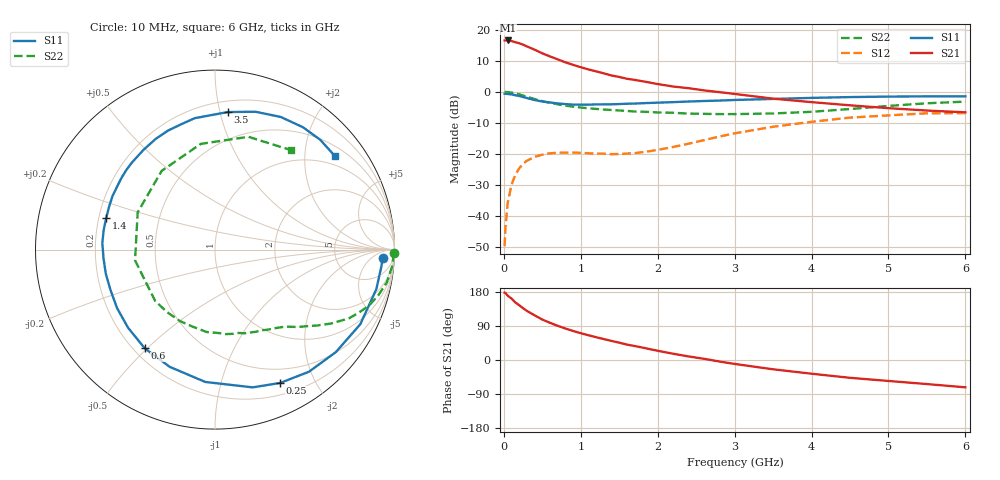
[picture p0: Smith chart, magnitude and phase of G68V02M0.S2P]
! SIEMENS Small Signal Semiconductors
! BFG193
! Si NPN RF Bipolar Junction Transistor in SOT223
! VCE = 8 V  IC = 2 mA
! Common Emitter S-Parameters:  August  1996
# GHz  S  MA  R  50
!  f  S11  S21  S12  S22
! GHz  MAG  ANG  MAG  ANG  MAG  ANG  MAG  ANG
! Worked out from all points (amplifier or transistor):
!   36 points, 10 MHz to 6 GHz, reference 50 ohm
!   highest |S21| = 16.5 dB at 50 MHz (marker M1)
!   |S21| within 3 dB of that: start of sweep to 402.1 MHz
!   unconditionally stable (mu >= 1): 1.376 GHz to 2.522 GHz
!   at 250 MHz: K = 0.17, MSG = 19.1 dB, |S12| = -23.1 dB
!   at 1.4 GHz: K = 1.02, MAG = 11.7 dB, |S12| = -20.0 dB
!   at 6 GHz: K = 0.94, MSG = 0.1 dB, |S12| = -6.8 dB
!   S11 on the Smith chart (normalised r, x): 10 MHz: 19, -14; 250 MHz: 0.33, -1.55; 600 MHz: 0.24, -0.49; 1.4 GHz: 0.23, +0.14; 3.5 GHz: 0.28, +1.06; 6 GHz: 0.74, +2.72
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0.01  0.9345 -2.8  6.709 177.8  0.0033 92.7  0.9971 -1.1
0.02  0.9321 -5.6  6.712 177.0  0.0064 86.3  0.9951 -2.2
0.05  0.9255 -13.8  6.713 169.8  0.0164 82.5  0.9909 -5.5
0.1  0.9101 -27.2  6.557 162.0  0.0321 75.4  0.9746 -10.8
0.15  0.8829 -40.3  6.29 151.9  0.0469 67.2  0.9446 -15.7
0.25  0.827 -63.9  5.748 136.6  0.07 55.3  0.8716 -24.0
0.3  0.7958 -74.7  5.39 129.6  0.0781 50.4  0.8384 -27.2
0.4  0.7394 -94.2  4.766 117.9  0.0902 41.4  0.7666 -32.5
0.5  0.7003 -111.1  4.164 106.7  0.0977 34.5  0.7093 -36.6
0.6  0.6752 -125.4  3.718 98.2  0.1029 29.8  0.6666 -39.8
0.7  0.6512 -138.1  3.334 90.2  0.1049 25.7  0.6323 -43.0
0.8  0.6355 -149.2  2.989 83.1  0.1053 22.7  0.6007 -45.7
0.9  0.6243 -158.8  2.721 76.6  0.1058 21.1  0.5783 -48.0
1.1  0.6231 -175.6  2.295 65.3  0.1031 19.3  0.5447 -54.1
1.4  0.6313 163.6  1.834 50.3  0.0996 20.7  0.5116 -63.4
1.6  0.6443 152.4  1.626 40.7  0.1017 24.4  0.4943 -70.6
2.2  0.6837 125.7  1.22 16.6  0.13 34.6  0.4615 -95.8
2.8  0.7241 104.7  0.991 -3.9  0.1909 33.4  0.4389 -127.8
3.5  0.7697 84.7  0.778 -24.5  0.2748 19.5  0.4495 -172.3
4.5  0.8248 63.6  0.608 -47.0  0.3856 -5.0  0.5299 124.1
5.5  0.8475 46.2  0.501 -63.5  0.4521 -34.5  0.6553 73.5
6  0.847 38.1  0.469 -72.1  0.4551 -50.3  0.6972 52.7
